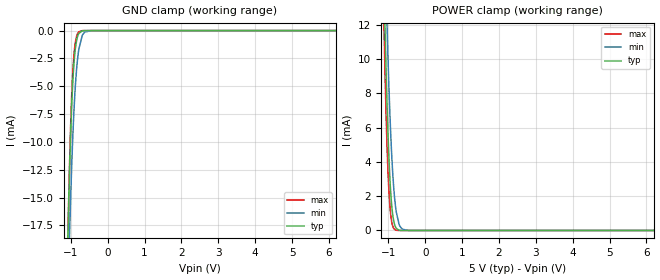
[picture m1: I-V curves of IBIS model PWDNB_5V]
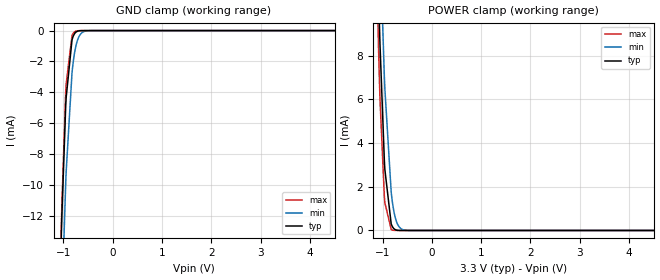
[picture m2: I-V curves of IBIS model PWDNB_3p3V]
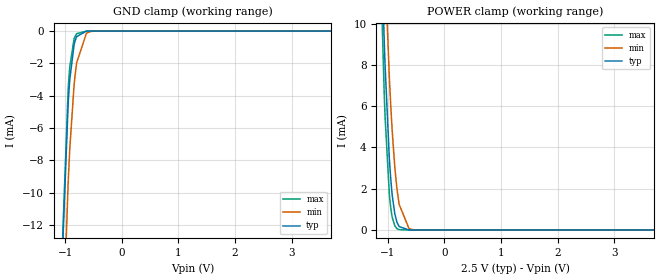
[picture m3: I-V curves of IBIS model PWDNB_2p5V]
| Texas Instruments Incorporated
| Low-noise 16-bit, 3-Channel AFE for Building Automation
| Marketing part#   Voltage Range   Package-type   #pins/pkg drawing
| LMP93601NHZ   1.65V - 5.5V   WQFN   24 / NHZ
[IBIS Ver]   4.1
[File name]   lmp93601.ibs
[File Rev]   1.0
[Date]   10/07/2013
[Source]   Model built from spectre simulations at:
   Texas Instruments Incorporated.
   Analog-eLab, HPA
   12500 TI Blvd
   Dallas, TX -75243
   For Support e-mail: elab_ibis@list.ti.com
[Notes]   Revision History
   Rev 1.0: 10/07/2013
   - Pullup/Pulldown non-monotonic for SDO output buffer
   - ccomp values are based on PVT settings:
   MIN: Low Voltage, High Temperature, Weak Process
   TYP: Nominal Voltage, Nominal Temperature, Nominal Process
   MAX: High Voltage, Low Temperature, Fast Process
   - C_comp although listed in numerical order of value are obtained from varying PVT conditions.
   For PVT conditions for each specific value, refer to the buffer description under respective [Model].
   IBIS model user is responsible for using appropriate C_comp to simulate for Signal Integrity.
[Disclaimer]  This model is designed as an aid for customers of Texas Instruments
 TI and its licensors and suppliers make no warranties, either expressed
 or implied, with respect to this  model, including the warranties of
 merchantability or fitness for a particular purpose.
 The model is provided solely on an "as is" basis. The entire risk as to
 its quality and performance is with the customer.
[Copyright] (C)Copyright 2013 Texas Instruments Incorporated.
   All rights reserved.
[Component]   LMP93601NHZ
[Manufacturer]  Texas Instruments Incorporated
[Package]   |24 Pin NHZ WQFN
|   typ   min   max
R_pkg   0   0   0
L_pkg   0   0   0
C_pkg   0   0   0
[Pin]   signal_name   model_name   R_pin   L_pin   C_pin
1   VCM   NC   0.08051  1.08157n  0.15544p
2   INP1   NC   0.06683  0.86950n  0.15680p
3   INN1   NC   0.06311  0.81306n  0.15181p
4   INP2   NC   0.06041  0.77284n  0.14864p
5   INN2   NC   0.06259  0.80525n  0.15210p
6   INP3   NC   0.07503  0.99550n  0.16648p
7   INN3   NC   0.08087  1.08717n  0.15306p
8   AGND   GND   0.10333  1.44227n  0.17005p
9   PWDNB   PWDNB   0.12401  1.76917n  0.21292p
10   RSTB   SYNC   0.11152  1.57059n  0.20710p
11   SYNC   SYNC   0.10332  1.44157n  0.19669p
12   XCLK   SYNC   0.10011  1.39257n  0.17476p
13   DRDYB   SDO   0.08422  1.14447n  0.15765p
14   SDI   SDI   0.08132  1.09856n  0.17389p
15   CSB   CSB   0.06699  0.87834n  0.15965p
16   IOGND   GND   0.05990  0.77344n  0.14999p
17   SCLK   SDI   0.06417  0.83618n  0.15565p
18   SDO   SDO   0.07730  1.03606n  0.16888p
19   IOVDD   POWER   0.08013  1.08067n  0.15287p
20   DGND   GND   0.10016  1.39377n  0.17127p
21   AGND   GND   0.10041  1.39647n  0.18896p
22   XCAP2   NC   0.10408  1.45340n  0.19437p
23   XCAP1   NC   0.11095  1.56167n  0.19698p
24   AVDD   POWER   0.10423  1.45637n  0.17143p
[Model Selector] SDO
SDO_1p8V   SDO OUTPUT, 1.8V SUPPLY
SDO_2p5V   SDO OUTPUT, 2.5V SUPPLY
SDO_3p3V   SDO OUTPUT, 3.3V SUPPLY
SDO_5V   SDO OUTPUT, 5V SUPPLY
[Model Selector] SDI
SDI_1p8V   SDI INPUT, 1.8V SUPPLY
SDI_2p5V   SDI INPUT, 2.5V SUPPLY
SDI_3p3V   SDI INPUT, 3.3V SUPPLY
SDI_5V   SDI INPUT, 5V SUPPLY
[Model Selector] CSB
CSB_1p8V   CSB INPUT, 1.8V SUPPLY
CSB_2p5V   CSB INPUT, 2.5V SUPPLY
CSB_3p3V   CSB INPUT, 3.3V SUPPLY
CSB_5V   CSB INPUT, 5V SUPPLY
[Model Selector] SYNC
SYNC_1p8V   SYNC INPUT, 1.8V SUPPLY
SYNC_2p5V   SYNC INPUT, 2.5V SUPPLY
SYNC_3p3V   SYNC INPUT, 3.3V SUPPLY
SYNC_5V   SYNC INPUT, 5V SUPPLY
[Model Selector] PWDNB
PWDNB_1p8V   PWDNB INPUT, 1.8V SUPPLY
PWDNB_2p5V   PWDNB INPUT, 2.5V SUPPLY
PWDNB_3p3V   PWDNB INPUT, 3.3V SUPPLY
PWDNB_5V   PWDNB INPUT, 5V SUPPLY
| Models and submodels in the file (20): PWDNB_5V (Input), PWDNB_3p3V (Input), PWDNB_2p5V (Input), PWDNB_1p8V (Input), CSB_5V (Input), CSB_3p3V (Input), CSB_2p5V (Input), CSB_1p8V (Input), SDI_5V (Input), SDI_3p3V (Input), SDI_2p5V (Input), SDI_1p8V (Input), SYNC_5V (Input), SYNC_3p3V (Input), SYNC_2p5V (Input), SYNC_1p8V (Input), SDO_5V (3-state), SDO_3p3V (3-state), SDO_2p5V (3-state), SDO_1p8V (3-state)
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|   (nom PVT)   (slow PVT)   (fast PVT)
|   Model PWDNB_5V
[Model]   PWDNB_5V
Model_type   Input
Vinl = 1.35
Vinh = 3.85
|   typ   min   max
|   (nom PVT)   (fast PVT)   (slow PVT)
C_comp   0.1436pF   0.1360pF   0.1525pF
[Model spec]
|subparameter
Vinl   1.5   1.35   1.65
Vinh   3.5   3.15   3.85
[Voltage Range]   5.0   4.5   5.5
[Temperature Range]   27   125   -25
[Power Clamp Reference]   5.0   4.5   5.5
[GND Clamp Reference]   0   0   0
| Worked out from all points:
|   GND clamp passes 1 mA (typ) near -0.85 V on its own axis
|   POWER clamp passes 1 mA (typ) near -0.89 V on its own axis
[GND Clamp]
|   Voltage   I(typ)   I(min)   I(max)
-5V       -931mA     -841.7mA   -990.9mA
-1.085V   -19.12mA   -24.53mA   -19.08mA
-1.07V    -16.98mA   -22.54mA   -16.71mA
-1.04V    -13.06mA   -18.79mA   -12.43mA
-1.025V   -11.31mA   -17.04mA   -10.55mA
-980mV    -6.906mA   -12.33mA   -5.968mA
-935mV    -3.84mA    -8.491mA   -2.991mA
-890mV    -1.94mA    -5.55mA    -1.317mA
-830mV    -668.1uA   -2.901mA   -359.3uA
-695mV    -26.7uA    -469.2uA   -7.095uA
-440mV    -371.4nA   -2.176uA   0A
9.985V    0A         0A         0A
[POWER Clamp]
|   Voltage   I(typ)   I(min)   I(max)
-5V       579.1mA    527.5mA    611.4mA
-1.13V    15.43mA    19.78mA    12.93mA
-1.115V   13.97mA    18.41mA    11.41mA
-1.085V   11.21mA    15.78mA    8.613mA
-1.04V    7.59mA     12.15mA    5.132mA
-1.01V    5.582mA    9.968mA    3.369mA
-965mV    3.248mA    7.121mA    1.579mA
-890mV    1.045mA    3.604mA    307.7uA
-800mV    173.6uA    1.289mA    18.8uA
-680mV    5.692uA    220.7uA    121.2nA
-455mV    0A         1.469uA    0A
9.985V    0A         0A         0A
|   Model PWDNB_3p3V
[Model]   PWDNB_3p3V
Model_type   Input
Vinl = .9
Vinh = 2.52
|   typ   min   max
|   (nom PVT)   (fast PVT)   (slow PVT)
C_comp   0.1436pF   0.1360pF   0.1525pF
[Model spec]
|subparameter
Vinl   0.99   0.9   1.08
Vinh   2.31   2.1   2.52
[Voltage Range]   3.3   3.0   3.6
[Temperature Range]   27   125   -25
[Power Clamp Reference]   3.3   3.0   3.6
[GND Clamp Reference]   0   0   0
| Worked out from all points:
|   GND clamp passes 1 mA (typ) near -0.84 V on its own axis
|   POWER clamp passes 1 mA (typ) near -0.86 V on its own axis
[GND Clamp]
|   Voltage   I(typ)   I(min)   I(max)
-3.3V     -526.6mA   -475.1mA   -563.8mA
-1.053V   -14.66mA   -20.34mA   -14.17mA
-1.043V   -13.41mA   -19.13mA   -12.81mA
-1.033V   -12.21mA   -17.95mA   -11.52mA
-953.7mV  -4.958mA   -9.976mA   -4.047mA
-943.8mV  -4.34mA    -9.17mA    -3.458mA
-825mV    -605.9uA   -2.736mA   -319.1uA
-785.4mV  -264.9uA   -1.684mA   -117.1uA
-745.8mV  -104.2uA   -992.6uA   -37.98uA
-646.8mV  -6.219uA   -211.1uA   -1.128uA
-468.6mV  -9.255nA   -4.518uA   0A
6.59V     0A         0A         0A
[POWER Clamp]
|   Voltage   I(typ)   I(min)   I(max)
-3.3V     323.2mA    295.8mA    340.5mA
-1.181V   20.82mA    24.71mA    18.6mA
-1.082V   10.98mA    15.56mA    8.388mA
-1.063V   9.324mA    13.92mA    6.763mA
-1.053V   8.542mA    13.13mA    6.018mA
-963.6mV  3.189mA    7.041mA    1.538mA
-953.7mV  2.79mA     6.49mA     1.273mA
-825mV    302.4uA    1.756mA    45.52uA
-805.2mV  195.7uA    1.376mA    22.75uA
-696.3mV  9.709uA    289.4uA    255.6nA
-528mV    22.07nA    9.496uA    0A
6.59V     0A         0A         0A
|   Model PWDNB_2p5V
[Model]   PWDNB_2p5V
Model_type   Input
Vinl = 0.675
Vinh = 1.925
|   typ   min   max
|   (nom PVT)   (fast PVT)   (slow PVT)
C_comp   0.1436pF   0.1360pF   0.1525pF
[Model spec]
|subparameter
Vinl   0.75   0.675   0.825
Vinh   1.75   1.575   1.925
[Voltage Range]   2.5   2.25   2.75
[Temperature Range]   27   125   -25
[Power Clamp Reference]   2.5   2.25   2.75
[GND Clamp Reference]   0   0   0
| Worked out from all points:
|   GND clamp passes 1 mA (typ) near -0.85 V on its own axis
|   POWER clamp passes 1 mA (typ) near -0.88 V on its own axis
[GND Clamp]
|   Voltage   I(typ)   I(min)   I(max)
-2.5V     -336.2mA   -303.6mA   -362.1mA
-1.045V   -13.68mA   -19.4mA    -13.1mA
-1.038V   -12.76mA   -18.5mA    -12.11mA
-947.5mV  -4.564mA   -9.466mA   -3.67mA
-940mV    -4.119mA   -8.873mA   -3.25mA
-917.5mV  -2.979mA   -7.242mA   -2.208mA
-842.5mV  -847.5uA   -3.346mA   -480.3uA
-835mV    -735.5uA   -3.073mA   -404.1uA
-797.5mV  -344.8uA   -1.962mA   -161uA
-625mV    -3.072uA   -142.4uA   -461.6nA
-520mV    -77.11nA   -15.71uA   -2.842nA
4.992V    0A         0A         0A
[POWER Clamp]
|   Voltage   I(typ)   I(min)   I(max)
-2.5V     204.2mA    188.6mA    214.4mA
-1.157V   18.25mA    22.37mA    15.88mA
-1.06V    9.115mA    13.71mA    6.563mA
-1.045V   7.958mA    12.53mA    5.472mA
-970mV    3.467mA    7.411mA    1.731mA
-947.5mV  2.56mA     6.16mA     1.126mA
-872.5mV  767.8uA    3.005mA    193.9uA
-835mV    372.6uA    1.977mA    63.34uA
-797.5mV  163.8uA    1.248mA    17.13uA
-625mV    848.8nA    80.83uA    8.785nA
-542.5mV  40.11nA    13.45uA    0A
4.992V    0A         0A         0A
